FUNCTION "DIVE" : VOID
TITLE =
VERSION : 0.1


VAR_TEMP
  zero : BOOL ;
END_VAR
BEGIN
NETWORK
TITLE =Produzione in corso
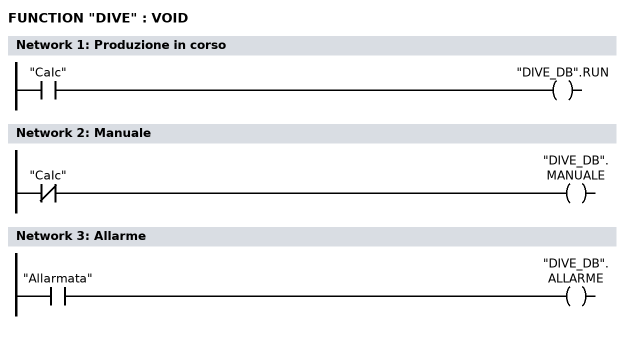
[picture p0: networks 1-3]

      U     "CaIc";
      =     "DIVE_DB".RUN;
NETWORK
TITLE =Manuale

      UN    "CaIc";
      =     "DIVE_DB".MANUALE;
NETWORK
TITLE =Allarme

      U     "Allarmata";
      =     "DIVE_DB".ALLARME;
NETWORK
TITLE =

      CLR   ;
      =     "ALWAYS_0";
      U     "ALWAYS_0";
      =     #zero;

NETWORK
TITLE =Mancato Carico
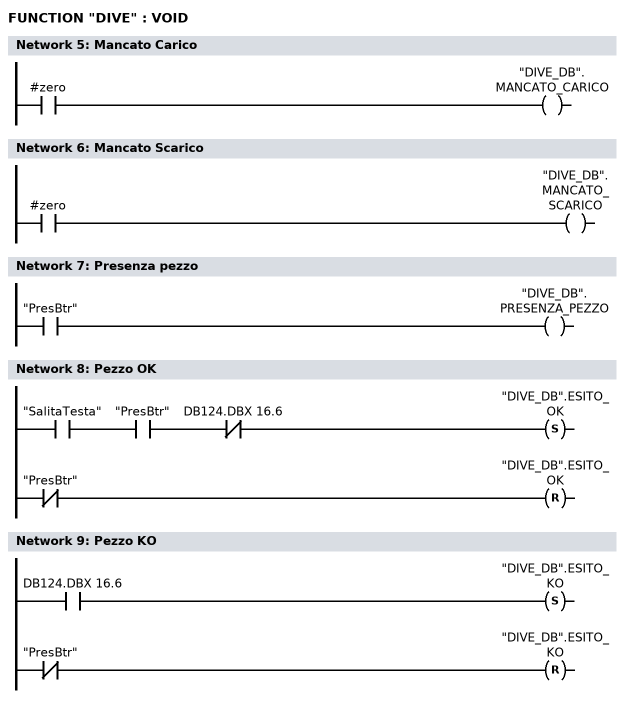
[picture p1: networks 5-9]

      U     #zero;
      =     "DIVE_DB".MANCATO_CARICO;
NETWORK
TITLE =Mancato Scarico

      U     #zero;
      =     "DIVE_DB".MANCATO_SCARICO;
NETWORK
TITLE =Presenza pezzo

      U     "PresBtr";
      =     "DIVE_DB".PRESENZA_PEZZO;
NETWORK
TITLE =Pezzo OK

      U     "SalitaTesta";
      U     "PresBtr";
      UN    DB124.DBX   16.6;
      S     "DIVE_DB".ESITO_OK;
      UN    "PresBtr";
      R     "DIVE_DB".ESITO_OK;
      NOP   0;
NETWORK
TITLE =Pezzo KO

      U     DB124.DBX   16.6;
      S     "DIVE_DB".ESITO_KO;
      UN    "PresBtr";
      R     "DIVE_DB".ESITO_KO;
      NOP   0;
NETWORK
TITLE =Fine Lavoro

      U(    ;
      U(    ;
      O     "SalitaTesta";
      O     DB124.DBX   16.6;
      )     ;
      S     "M254.3";
      UN    "PresBtr";
      R     "M254.3";
      U     "M254.3";
      )     ;
      L     S5T#500MS;
      SE    T     15;
      NOP   0;
      NOP   0;
      NOP   0;
      U     T     15;
      =     "DIVE_DB".FINE_LAVORO;
NETWORK
TITLE =Inizio Pallet
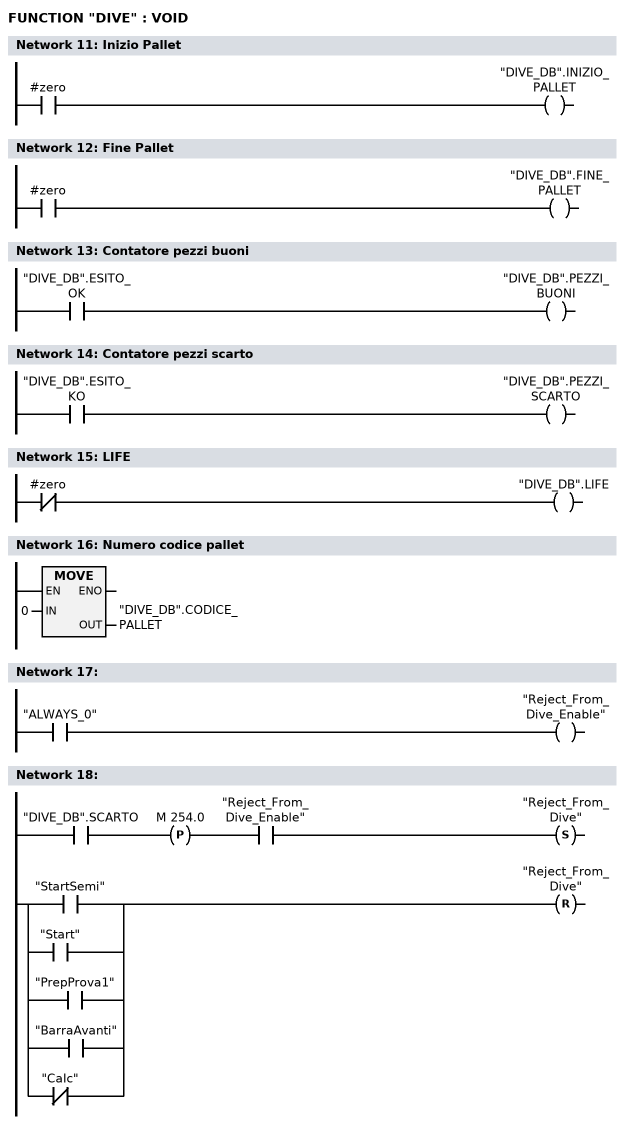
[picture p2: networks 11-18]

      U     #zero;
      =     "DIVE_DB".INIZIO_PALLET;
NETWORK
TITLE =Fine Pallet

      U     #zero;
      =     "DIVE_DB".FINE_PALLET;
NETWORK
TITLE =Contatore pezzi buoni

      U     "DIVE_DB".ESITO_OK;
      =     "DIVE_DB".PEZZI_BUONI;
NETWORK
TITLE =Contatore pezzi scarto

      U     "DIVE_DB".ESITO_KO;
      =     "DIVE_DB".PEZZI_SCARTO;
NETWORK
TITLE =LIFE

      UN    #zero;
      =     "DIVE_DB".LIFE;
NETWORK
TITLE =Numero codice pallet

      L     0;
      T     "DIVE_DB".CODICE_PALLET;
      NOP   0;
NETWORK
TITLE =

      U     "ALWAYS_0";
      =     "Reject_From_Dive_Enable";
NETWORK
TITLE =

      U     "DIVE_DB".SCARTO;
      FP    M    254.0;
      U     "Reject_From_Dive_Enable";
      S     "Reject_From_Dive";
      U(    ;
      O     "StartSemi";
      O     "Start";
      O     "PrepProva1";
      O     "BarraAvanti";
      ON    "CaIc";
      )     ;
      R     "Reject_From_Dive";
      NOP   0;
END_FUNCTION

